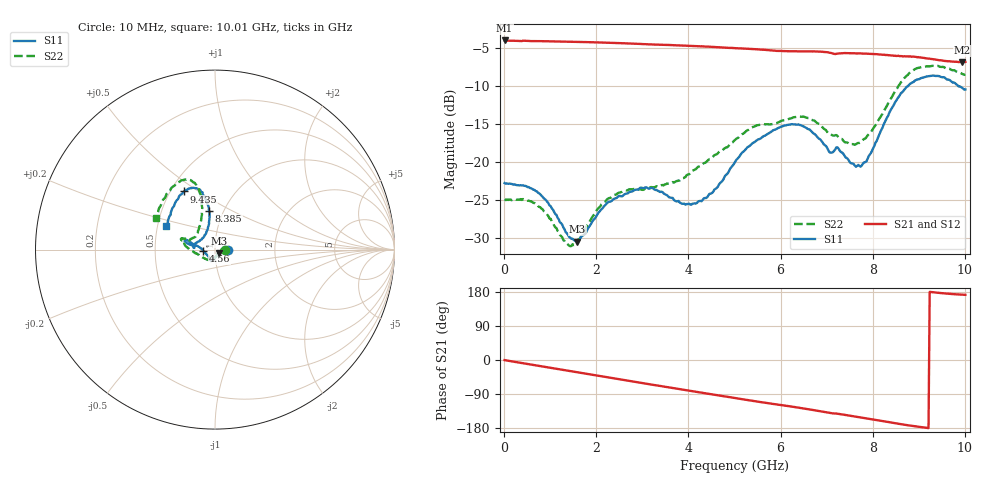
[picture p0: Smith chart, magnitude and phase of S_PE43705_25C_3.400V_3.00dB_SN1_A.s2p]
! Device ID: PE43705
! Serial: 1
! Insertion: A
! Impedance: 50 ohm
! Temp: 25C
! VDD: 3.400V
! Attenuation Step: 3.00dB
#  Hz  S  RI  R  50
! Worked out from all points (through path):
!   401 points, 10 MHz to 10.01 GHz, reference 50 ohm
!   highest |S21| = -4.01 dB at 10 MHz (marker M1); lowest = -6.9 dB at 9.935 GHz (marker M2)
!   group delay of S21, straight-line fit = 53.5 ps
!   lowest |S11| = -30.5 dB at 1.585 GHz (marker M3), VSWR 1.06, Z = 52.1 - j2.23 ohm
!   |S11| at or under -10 dB: start of sweep to 8.767 GHz; 9.851 GHz to end of sweep
!   |S22| runs from -31.1 to -7.4 dB; largest |S21 - S12| = 0.0052
!   S11 on the Smith chart (normalised r, x): 10 MHz: 1.16, -0.00; 4.56 GHz: 0.88, -0.01; 8.385 GHz: 0.86, +0.39; 9.435 GHz: 0.58, +0.44; 10.01 GHz: 0.56, +0.16
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1e7  0.0725 -0.000381  0.63 -0.00309  0.6307 -0.00286  0.0567 -0.000105
7.35e8  0.0607 0.0153  0.6014 -0.1638  0.6016 -0.1635  0.0491 0.0143
1.36e9  0.0329 -0.00831  0.5467 -0.29  0.5467 -0.2897  0.0267 -0.0113
1.585e9  0.0207 -0.0214  0.5193 -0.3315  0.5195 -0.3315  0.0168 -0.0249
1.685e9  0.0162 -0.0283  0.5069 -0.3492  0.5068 -0.3491  0.0113 -0.0312
2.31e9  -0.00678 -0.0543  0.4129 -0.4461  0.4131 -0.4457  -0.0145 -0.056
2.985e9  -0.0204 -0.0643  0.2917 -0.5211  0.2921 -0.5209  -0.0322 -0.057
3.36e9  -0.023 -0.0596  0.2209 -0.548  0.2215 -0.5476  -0.0386 -0.0571
4.01e9  -0.0394 -0.0356  0.0918 -0.573  0.0921 -0.5724  -0.0711 -0.0424
4.56e9  -0.0651 -0.00757  -0.0169 -0.5696  -0.0156 -0.5694  -0.1083 -0.0215
5.01e9  -0.0977 0.0201  -0.101 -0.5516  -0.1006 -0.5519  -0.1394 2.46e-05
6.01e9  -0.1616 0.0537  -0.2593 -0.4701  -0.2572 -0.4709  -0.1797 0.0478
6.685e9  -0.1531 0.0335  -0.3543 -0.3986  -0.3544 -0.3983  -0.1777 0.0628
7.085e9  -0.1137 0.0164  -0.3999 -0.3356  -0.4003 -0.3365  -0.1427 0.052
7.71e9  -0.0672 0.0659  -0.4534 -0.2498  -0.4523 -0.2507  -0.0978 0.0903
7.91e9  -0.0483 0.0975  -0.4665 -0.2167  -0.4665 -0.2195  -0.0885 0.1233
8.36e9  -0.0312 0.2087  -0.4843 -0.1381  -0.4831 -0.1401  -0.0728 0.2414
8.385e9  -0.0324 0.2161  -0.4845 -0.1328  -0.4825 -0.136  -0.0731 0.2483
8.86e9  -0.0802 0.324  -0.4898 -0.0522  -0.4869 -0.0545  -0.124 0.3769
9.435e9  -0.1734 0.3237  -0.4667 0.0231  -0.4659 0.0236  -0.2192 0.3649
9.935e9  -0.2621 0.1616  -0.4497 0.0594  -0.451 0.0588  -0.3168 0.2093
1.001e10  -0.2706 0.1292  -0.4506 0.064  -0.452 0.0625  -0.3293 0.1786
